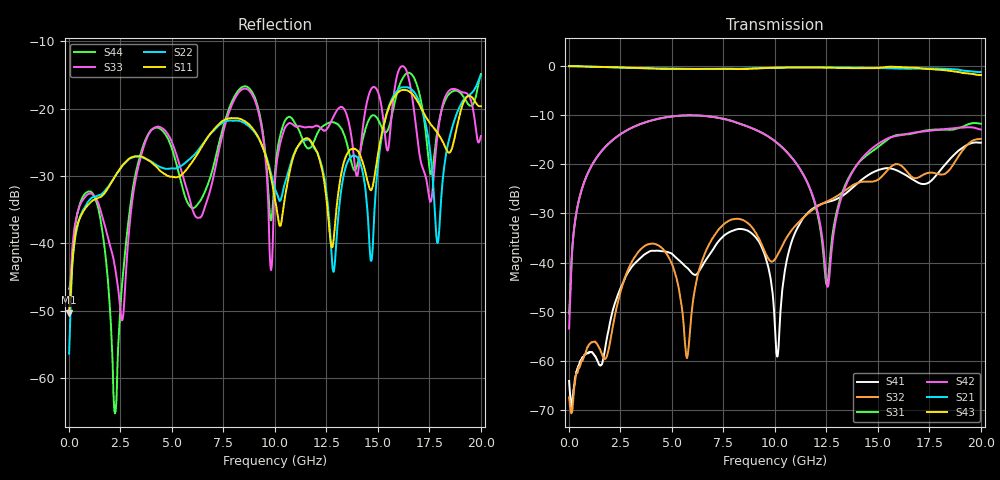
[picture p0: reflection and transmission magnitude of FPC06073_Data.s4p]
!Agilent Technologies,N5225A,MY51451324,A.10.20.03
!Agilent N5225A: A.10.20.03
!Date: Thursday, February 12, 2015 14:05:36
!Correction: S11(Full 4 Port(1,2,3,4))
!S12(Full 4 Port(1,2,3,4))
!S13(Full 4 Port(1,2,3,4))
!S14(Full 4 Port(1,2,3,4))
!S21(Full 4 Port(1,2,3,4))
!S22(Full 4 Port(1,2,3,4))
!S23(Full 4 Port(1,2,3,4))
!S24(Full 4 Port(1,2,3,4))
!S31(Full 4 Port(1,2,3,4))
!S32(Full 4 Port(1,2,3,4))
!S33(Full 4 Port(1,2,3,4))
!S34(Full 4 Port(1,2,3,4))
!S41(Full 4 Port(1,2,3,4))
!S42(Full 4 Port(1,2,3,4))
!S43(Full 4 Port(1,2,3,4))
!S44(Full 4 Port(1,2,3,4))
!S4P File: Measurements: <S11,S12,S13,S14>,
!<S21,S22,S23,S24>,
!<S31,S32,S33,S34>,
!<S41,S42,S43,S44>:
# Hz S  dB  R 50
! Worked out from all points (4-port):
!   2000 points, 10 MHz to 20 GHz, reference 50 ohm
!   strongest paths, dB at 10 MHz, 5.01 GHz, 10.01 GHz, 15.01 GHz, 20 GHz:
!     S43: 0.0, -0.6, -0.4, -0.4, -1.8
!     S21: -0.1, -0.6, -0.4, -0.4, -1.2
!     S42: -53.4, -10.3, -15.3, -15.9, -12.9
!     S31: -50.4, -10.3, -15.3, -16.5, -11.8
!     S32: -67.5, -40.4, -39.3, -23.1, -14.8
!     S41: -64.1, -38.3, -53.7, -21.2, -15.6
!   lowest |S11| = -50.3 dB at 10 MHz (marker M1), VSWR 1.01, Z = 50.1 + j0.285 ohm
!   |S11| at or under -10 dB: start of sweep to end of sweep
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1e7  -50.28 68.1  -0.04 -0.9  -55.91 66.7  -62.00 -127.1
     -0.05 -0.9  -56.35 104.8  -62.46 150.5  -49.57 82.0
     -50.41 115.7  -67.45 -47.0  -50.29 15.5  -0.04 -0.9
     -64.10 154.0  -53.44 105.4  -0.04 -0.9  -46.72 132.9
1.28e9  -33.43 33.9  -0.16 -30.2  -19.06 59.7  -59.29 159.1
        -0.16 -30.1  -33.07 27.6  -56.30 150.6  -19.06 59.6
        -19.06 59.7  -56.13 150.0  -33.08 34.1  -0.16 -30.6
        -59.06 158.1  -19.06 59.6  -0.15 -30.6  -33.39 31.4
2.24e9  -30.02 31.5  -0.29 -51.8  -14.68 38.0  -48.25 -164.1
        -0.29 -51.8  -30.04 28.2  -50.68 -161.9  -14.68 37.8
        -14.69 38.0  -50.65 -161.8  -43.60 -53.6  -0.28 -52.6
        -48.20 -164.0  -14.68 37.8  -0.28 -52.5  -65.12 150.5
3.06e9  -27.18 16.0  -0.40 -70.0  -12.56 19.7  -40.87 156.3
        -0.40 -70.0  -27.26 8.8  -39.86 155.1  -12.56 19.4
        -12.56 19.7  -39.81 155.1  -34.03 13.9  -0.39 -71.1
        -40.82 156.5  -12.56 19.4  -0.39 -71.1  -32.74 -11.6
1.012e10  -35.49 -66.3  -0.35 132.5  -15.72 -136.9  -58.61 4.6
          -0.34 132.5  -32.79 156.2  -38.59 122.0  -15.72 -138.3
          -15.71 -136.9  -38.55 122.0  -27.31 -1.2  -0.35 129.1
          -59.15 4.7  -15.71 -138.3  -0.35 129.1  -26.19 69.1
1.19e10  -25.61 4.7  -0.27 90.1  -27.44 -173.1  -28.89 6.8
         -0.26 90.2  -25.82 3.6  -29.08 12.3  -27.16 -173.2
         -27.43 -173.2  -29.07 12.3  -22.64 39.0  -0.31 85.9
         -28.86 6.9  -27.15 -173.3  -0.31 85.9  -24.84 -55.2
2e10  -19.62 21.6  -1.24 -104.5  -11.77 160.5  -15.63 153.6
      -1.23 -104.4  -15.10 43.6  -14.85 154.4  -12.94 155.8
      -11.76 160.5  -14.83 154.3  -24.06 61.8  -1.85 -110.8
      -15.60 153.6  -12.92 155.8  -1.85 -110.8  -14.88 66.4
